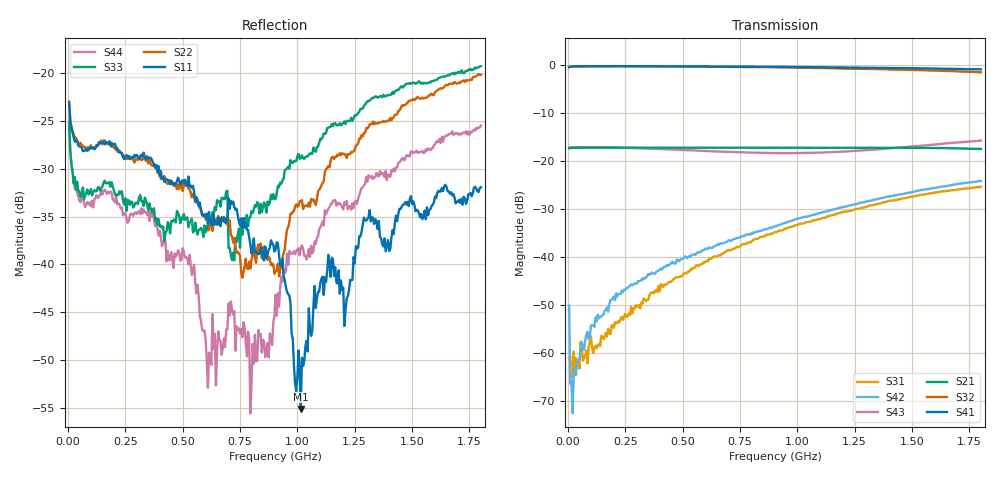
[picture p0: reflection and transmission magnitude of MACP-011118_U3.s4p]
!Agilent Technologies,E5071C,MY46110647,A.11.31
!Date: Thu Jan 18 12:40:40 2024 DD
!Data & Calibration Information:
!MACP-011118 soldered onto PT-0003645 with F connectors, Calibration PT-0003645-TRL. Port1 (pin3) Port2 (pin1) Port3 (pin6) Port4 (pin4)
!Freq	S11:SOLT4(ON)	S12:SOLT4(ON)	S13:SOLT4(ON)	S14:SOLT4(ON)
!	S21:SOLT4(ON)	S22:SOLT4(ON)	S23:SOLT4(ON)	S24:SOLT4(ON)
!	S31:SOLT4(ON)	S32:SOLT4(ON)	S33:SOLT4(ON)	S34:SOLT4(ON)
!	S41:SOLT4(ON)	S42:SOLT4(ON)	S43:SOLT4(ON)	S44:SOLT4(ON)
!PortZ  Port1:75+j0  Port2:75+j0  Port3:75+j0  Port4:75+j0
!Above PortZ is port z conversion or system Z0 setting when saving the data.
!When reading, reference impedance value at option line is always used.
# Hz S MA R 75
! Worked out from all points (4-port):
!   360 points, 5 MHz to 1.8 GHz, reference 75 ohm
!   strongest paths, dB at 5 MHz, 455 MHz, 905 MHz, 1.355 GHz, 1.8 GHz:
!     S41: -0.5, -0.4, -0.5, -0.7, -1.0
!     S32: -0.5, -0.4, -0.5, -0.9, -1.6
!     S21: -17.4, -17.3, -17.3, -17.3, -17.5
!     S43: -17.2, -17.6, -18.4, -17.6, -15.8
!     S42: -50.1, -40.9, -33.6, -27.8, -24.2
!     S31: -61.0, -44.9, -34.8, -28.9, -25.4
!   lowest |S11| = -55.1 dB at 1.015 GHz (marker M1), VSWR 1.00, Z = 74.8 + j0.0966 ohm
!   |S11| at or under -10 dB: start of sweep to end of sweep
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5000000  0.06985 147.0  0.1351 -178.0  0.00147 50.5  0.9454 2.2
         0.1354 -177.3  0.071 148.2  0.9452 2.2  0.0007152 -57.6
         0.0008894 -106.4  0.9426 2.2  0.05472 134.0  0.1381 1.7
         0.944 2.3  0.003139 -97.3  0.1374 1.8  0.05881 136.1
2e7  0.0489 164.5  0.1364 179.5  0.0004523 -140.4  0.9556 0.4
     0.1364 179.6  0.04953 164.5  0.9556 0.3  0.0005268 -136.3
     0.0005567 -145.2  0.9568 0.3  0.03013 157.2  0.1383 0.4
     0.9555 0.4  0.000238 -153.8  0.1385 0.3  0.03062 155.1
2.1e8  0.04055 172.2  0.137 164.4  0.002069 148.3  0.9636 -5.6
       0.1374 164.3  0.03952 162.1  0.9633 -6.1  0.003581 102.5
       0.002096 151.6  0.963 -6.1  0.02293 153.4  0.1371 -3.1
       0.9634 -5.7  0.004215 94.3  0.1372 -3.1  0.02281 167.7
7.95e8  0.01275 173.3  0.1371 121.2  0.01363 103.2  0.9519 -22.2
        0.1372 121.2  0.009522 51.1  0.9445 -24.0  0.01689 80.4
        0.01419 109.6  0.9455 -24.0  0.01771 -17.7  0.1219 -5.0
        0.9522 -22.2  0.01751 78.6  0.1219 -4.9  0.001667 -122.1
1.015e9  0.001756 158.4  0.137 105.3  0.02099 87.8  0.9436 -28.4
         0.1368 105.4  0.0215 -24.2  0.9286 -30.9  0.02366 71.6
         0.02236 93.1  0.9296 -30.9  0.03593 -52.9  0.1204 -1.8
         0.9437 -28.4  0.02569 70.5  0.1208 -1.8  0.01227 -72.6
1.135e9  0.01122 -86.9  0.1366 96.7  0.02527 80.6  0.9381 -31.8
         0.1365 96.8  0.03276 -54.2  0.9176 -34.6  0.02839 67.3
         0.02652 84.9  0.9188 -34.6  0.05182 -70.0  0.1225 0.1
         0.9383 -31.8  0.03032 66.0  0.1231 0.0  0.01951 -86.0
1.8e9  0.02532 -133.7  0.133 45.9  0.05265 34.2  0.8926 -50.7
       0.133 45.7  0.09789 -113.4  0.8304 -54.7  0.05823 28.8
       0.05386 35.5  0.8322 -54.8  0.1087 -107.4  0.1618 -0.7
       0.8932 -50.8  0.06166 28.9  0.1622 -0.6  0.05313 -110.1
